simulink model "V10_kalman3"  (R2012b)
settings: Solver=FixedStepDiscrete  StartTime=0.0  StopTime=20  FixedStep=0.1  RelTol=1e-3
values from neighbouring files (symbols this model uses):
  Ts = 0.1    [V2_4_tdomain.m]    (also in V2_6_UTFDiskretizierung.m; V2_7_multiZ.m; DBDisk.m = 0.02; DBDisk2.m = 0.02)
undefined symbols (not defined in the file or in its folder): r1, r2, ro, xo
libraries: simulink x2

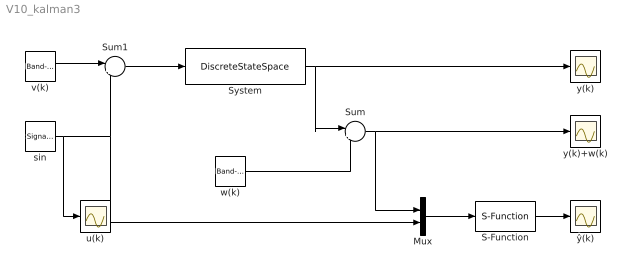
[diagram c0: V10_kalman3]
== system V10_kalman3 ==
  Mux : Mux  Inputs=2
  S-Function : S-Function  FunctionName=kalman3  Parameters=Ts,xo,ro,r1,r2  SFunctionDeploymentMode=off  EnableBusSupport=off
  Sum : Sum  Inputs=|++
  Sum1 : Sum  Inputs=|++
  System : DiscreteStateSpace  A=0.5  D=0  SampleTime=0.1
  sin : SignalGenerator
  u(k) : Scope
  v(k) : simulink/Sources/Band-Limited White Noise  Cov=[0.01]  Ts=0.1  seed=[23341]
  w(k) : simulink/Sources/Band-Limited White Noise  Cov=[0.1]  Ts=0.1  seed=[23341]
  y(k) : Scope
  y(k)+w(k) : Scope
  ŷ(k) : Scope
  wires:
  System/1 -> y(k)/1, Sum/1
  w(k)/1 -> Sum/2
  Sum/1 -> y(k)+w(k)/1, Mux/1
  S-Function/1 -> ŷ(k)/1
  v(k)/1 -> Sum1/1
  sin/1 -> u(k)/1, Sum1/2, Mux/2
  Sum1/1 -> System/1
  Mux/1 -> S-Function/1
